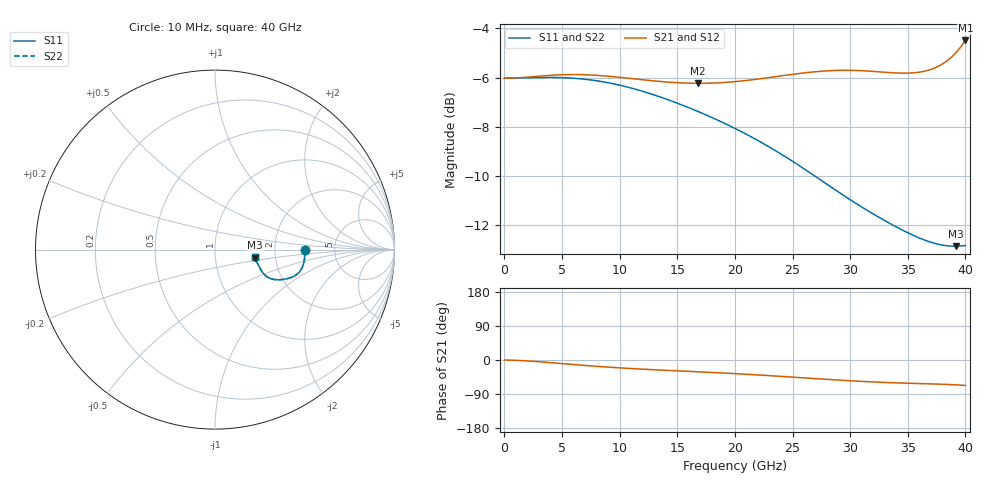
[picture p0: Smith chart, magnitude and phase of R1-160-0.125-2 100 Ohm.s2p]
!version-1
!date-09.2020
# MHz S RI R 50
!Freq ReS11 ImS11 ReS21 ImS21 ReS12 ImS12 ReS22 ImS22
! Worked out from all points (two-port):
!   101 points, 10 MHz to 40 GHz, reference 50 ohm
!   highest |S21| = -4.49 dB at 40 GHz (marker M1); lowest = -6.2 dB at 16.81 GHz (marker M2)
!   |S21| within 3 dB of the highest: start of sweep to end of sweep
!   lowest |S11| = -12.9 dB at 39.21 GHz (marker M3), VSWR 1.59, Z = 78.3 - j7.36 ohm
!   |S11| at or under -10 dB: 26.92 GHz to end of sweep
!   |S22| runs from -12.9 to -6.0 dB; largest |S21 - S12| = 0
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10  0.5 -7.49e-06  0.5 -4.35e-05  0.5 -4.35e-05  0.5 -7.49e-06
1210  0.5 -0.00625  0.5006 -0.0107  0.5006 -0.0107  0.5 -0.00625
2410  0.5004 -0.0203  0.5022 -0.0297  0.5022 -0.0297  0.5004 -0.0203
4810  0.4977 -0.0585  0.5013 -0.0795  0.5013 -0.0795  0.4977 -0.0585
6810  0.4894 -0.0904  0.493 -0.1222  0.493 -0.1222  0.4894 -0.0904
8410  0.479 -0.112  0.4821 -0.1524  0.4821 -0.1524  0.479 -0.112
10010  0.4659 -0.129  0.4692 -0.1777  0.4692 -0.1777  0.4659 -0.129
11610  0.451 -0.1417  0.4557 -0.1986  0.4557 -0.1986  0.451 -0.1417
13610  0.4305 -0.1528  0.4396 -0.2205  0.4396 -0.2205  0.4305 -0.1528
16810  0.395 -0.1633  0.4175 -0.2525  0.4175 -0.2525  0.395 -0.1633
20010  0.3575 -0.1678  0.3977 -0.2892  0.3977 -0.2892  0.3575 -0.1678
23610  0.3152 -0.1631  0.3715 -0.3399  0.3715 -0.3399  0.3152 -0.1631
26810  0.2823 -0.1455  0.3391 -0.387  0.3391 -0.387  0.2823 -0.1455
28410  0.2689 -0.1319  0.3196 -0.4073  0.3196 -0.4073  0.2689 -0.1319
30010  0.2579 -0.1164  0.2989 -0.4235  0.2989 -0.4235  0.2579 -0.1164
31610  0.2488 -0.1001  0.2788 -0.4348  0.2788 -0.4348  0.2488 -0.1001
33610  0.2388 -0.0806  0.2572 -0.4435  0.2572 -0.4435  0.2388 -0.0806
35610  0.2301 -0.0639  0.2421 -0.4519  0.2421 -0.4519  0.2301 -0.0639
37210  0.2249 -0.0536  0.2354 -0.4666  0.2354 -0.4666  0.2249 -0.0536
38410  0.2231 -0.0478  0.2332 -0.4892  0.2332 -0.4892  0.2231 -0.0478
39210  0.2233 -0.0445  0.2325 -0.5137  0.2325 -0.5137  0.2233 -0.0445
40000  0.2247 -0.041  0.2318 -0.5492  0.2318 -0.5492  0.2247 -0.041
